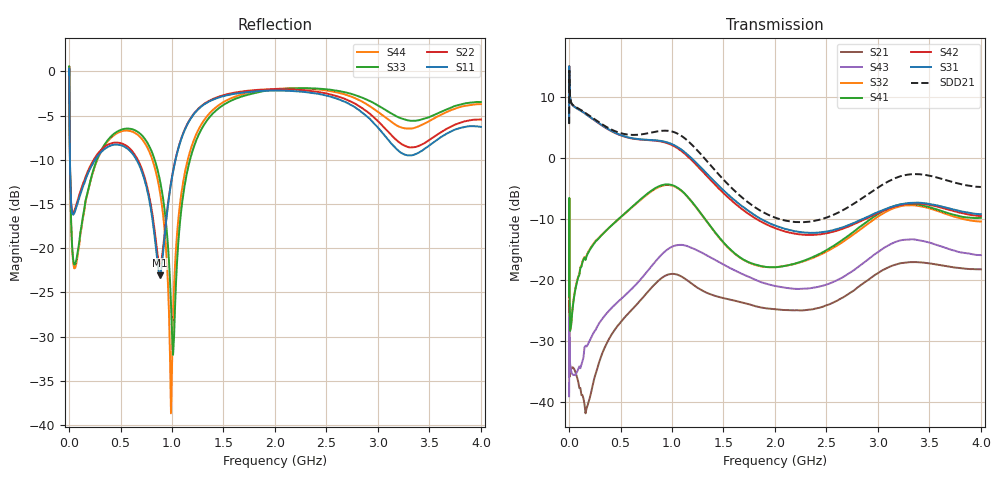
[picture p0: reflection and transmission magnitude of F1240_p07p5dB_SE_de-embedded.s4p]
! Integrated Device Technology
! Corporate Headquarters
! 6024 Silver Creek Valley Road
! San Jose, CA 95138  USA
! Phone:  1-408-284-8200
! Toll Free:  1-800-223-1366
! Webpage:  http://www.idt.com/
! Timing and RF Division
! 515 Groton Road, Suite 102
! Westford, MA 01886-6024
! Device:  F1240
! Description: Dual Intermediate Frequency Digital Variable Gain Amplifier
! Frequency:  10.0 -  500.00 MHz
! Package:  5x5 mm QFN Plastic Package: 32 pin
! Ports:  8 RF, 20 DC
!  Pin  1  = GA3 / Data  Pin 17  = RF OUT_B+
!  Pin  2  = GA4 / CLK  Pin 18  = RF OUT_B-
!  Pin  3  = GA5  Pin 19  = STBY_B
!  Pin  4  = VMODE  Pin 20  = Ground
!  Pin  5  = No Connect  Pin 21  = Ground
!  Pin  6  = GB5  Pin 22  = STB_A
!  Pin  7  = GB4  Pin 23  = RF OUT_A-  = Port 4
!  Pin  8  = GB3  Pin 24  = RF OUT_A+  = Port 3
!  Pin  9  = GB2  Pin 25  = GA0
!  Pin 10  = GB1  Pin 26  = ISET_A
!  Pin 11  = RF IN_B+  Pin 27  = VCC
!  Pin 12  = RF IN_B-  Pin 28  = Ground
!  Pin 13  = Ground  Pin 29  = RF IN_A-  = Port 2
!  Pin 14  = VCC  Pin 30  = RF IN_A+  = Port 1
!  Pin 15  = ISET_B  Pin 31  = GA1
!  Pin 16  = GB0  Pin 32  = GA2 / CSb
! Gain  = +19.5 dB
! State  = 1
! Voltage  = +5.00 V
! Current  = 85.292 mA (one channel only)
! Temperture  =  +25 C
! Test Date  =  2017-10-18
! Board  =  EB4031
! Data:  The device was measured on a custom evaluation board which has
!  individual transmission lines to the RF pins.  Data was collected
!  using a calibrated network analyzer.  The evaluation board was
!  de-embedded using Automatic Fixture Removal.
!  The reference plane is the edge of the package pin.
!  Only Channel A was measured.
!  This data is in single-ended operation.  If your needs are balanced
!  or differential S-parameters then this file needs to be used a
!  linear simulator.
! File Date:  2017-11-10  MJV
! Note:
!  Integrated Device Technology supplies this data as a sample of measured
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# Hz S dB R 100
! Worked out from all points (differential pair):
!   410 points, 500 kHz to 4 GHz, reference 100 ohm
!   strongest paths, dB at 500 kHz, 930 MHz, 1.96 GHz, 2.98 GHz, 4 GHz:
!     S31: 5.9, 2.7, -10.8, -9.0, -9.2
!     S42: 5.9, 2.6, -11.2, -9.2, -9.5
!     S41: -22.6, -4.3, -17.9, -9.4, -9.8
!     S32: -22.9, -4.4, -17.9, -9.8, -10.4
!     S43: -39.1, -15.3, -20.8, -15.7, -15.9
!     S21: -25.2, -19.3, -24.7, -19.1, -18.2
!   taken as a pair (ports 1,2 in; 3,4 out), SDD21 dB: 5.6, 4.5, -9.5, -5.1, -4.7
!   lowest |S11| = -23.1 dB at 880 MHz (marker M1), VSWR 1.15, Z = 111 + j9.55 ohm
!   |S11| at or under -10 dB: 8.743 MHz to 253.1 MHz (244.4 MHz wide, 187 % of centre); 655.2 MHz to 1.034 GHz (378.7 MHz wide, 44.8 % of centre)
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500000  -0.41 -5.6  -25.26 -5.6  -27.15 83.0  -57.64 71.9
        -25.24 -5.5  -0.41 -5.5  -58.02 68.7  -27.16 84.1
        5.90 -105.1  -22.88 -87.0  -0.50 1.5  -39.08 -93.1
        -22.62 -86.9  5.87 -103.9  -39.05 -93.5  -0.51 3.8
3000000  -2.36 -60.9  -30.92 -82.8  -15.30 27.6  -52.87 -53.2
         -31.05 -82.2  -2.32 -60.9  -52.65 -54.5  -15.31 27.8
         14.25 178.1  -11.38 146.6  -1.82 -56.4  -26.98 -176.3
         -11.53 146.3  14.25 178.4  -26.94 -176.3  -1.88 -56.2
3e7  -16.06 -120.3  -34.26 -8.9  -15.49 -7.6  -48.42 63.4
     -34.28 -9.1  -15.86 -120.3  -48.21 64.1  -15.48 -7.5
     8.75 162.4  -25.24 57.3  -19.86 -113.3  -35.62 157.1
     -25.44 56.9  8.78 162.4  -35.37 157.2  -20.14 -113.7
2e8  -11.13 -144.2  -39.84 19.9  -16.95 -49.7  -34.32 23.9
     -39.38 21.5  -10.85 -144.9  -34.30 24.6  -16.96 -49.8
     6.77 110.1  -14.98 8.7  -12.65 -110.5  -30.30 99.5
     -15.09 8.3  6.76 109.5  -29.93 98.4  -12.77 -109.4
8.8e8  -23.06 37.4  -20.19 -87.2  -16.01 172.8  -26.09 -136.9
       -19.93 -92.1  -21.92 39.5  -26.28 -129.9  -16.25 172.2
       2.84 -62.7  -4.70 -170.6  -12.17 134.8  -16.88 -70.3
       -4.58 -174.1  2.75 -64.3  -16.16 -72.4  -13.46 135.2
1.2e9  -5.03 -112.5  -20.09 -177.8  -18.24 84.3  -25.38 148.9
       -20.69 178.2  -4.97 -112.1  -24.90 155.7  -18.83 83.3
       -0.20 -157.0  -7.35 77.1  -8.97 -99.0  -15.26 -169.0
       -7.31 72.3  -0.50 -158.8  -14.79 -171.3  -8.16 -103.4
4e9  -6.28 -149.8  -18.35 86.3  -20.20 -68.5  -21.49 -48.2
     -18.24 85.6  -5.44 -147.6  -22.46 -28.5  -21.72 -61.2
     -9.21 23.9  -10.40 -90.9  -3.47 -140.1  -17.11 80.7
     -9.80 -105.5  -9.51 31.4  -15.91 58.4  -3.70 -147.8
